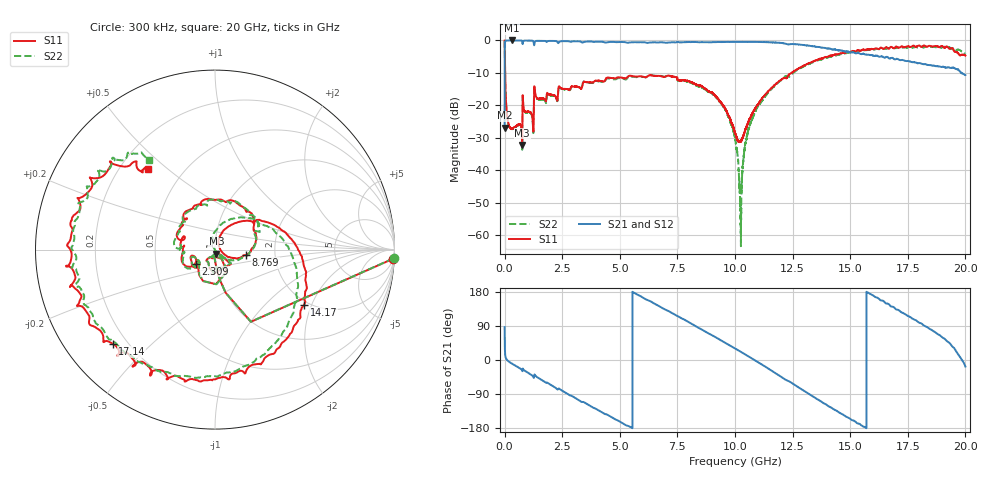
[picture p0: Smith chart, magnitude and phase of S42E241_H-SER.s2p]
! Created Wed Nov 25 22:07:44 2020
# khz S ma R 50
! 2 Port Network Data from SP1.SP block
! freq  magS11  angS11  magS21  angS21  magS12  angS12  magS22  angS22
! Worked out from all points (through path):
!   20001 points, 300 kHz to 20 GHz, reference 50 ohm
!   highest |S21| = -0.02 dB at 315.3 MHz (marker M1); lowest = -26.9 dB at 300 kHz (marker M2)
!   group delay of S21, straight-line fit = 97.6 ps
!   lowest |S11| = -32.2 dB at 763.3 MHz (marker M3), VSWR 1.05, Z = 50.8 - j2.36 ohm
!   |S11| at or under -10 dB: 20.12 MHz to 12.46 GHz (12.44 GHz wide, 199 % of centre)
!   |S22| runs from -63.4 to 0.0 dB; largest |S21 - S12| = 0.013
!   S11 on the Smith chart (normalised r, x): 300 kHz: 6, -38; 2.309 GHz: 0.80, -0.13; 8.769 GHz: 1.41, -0.09; 14.17 GHz: 1.90, -1.76; 17.14 GHz: 0.15, -0.38; 20 GHz: 0.32, +0.43
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300  0.9924 -3.0  0.04493 86.6  0.04459 86.7  0.9959 -2.8
103300  0.07189 -88.1  0.9948 0.2  0.9951 0.2  0.07176 -88.2
315300  0.04367 -96.5  0.9973 -9.4  0.9962 -9.5  0.04313 -96.8
763300  0.02454 -71.0  0.9798 -27.8  0.9799 -27.8  0.0206 -72.9
1370300  0.1345 -133.6  0.981 -43.4  0.9811 -43.4  0.1329 -131.8
2309300  0.1336 -144.3  0.9204 -77.8  0.9211 -77.8  0.1328 -140.0
3334300  0.1801 160.5  0.9443 -110.5  0.9444 -110.5  0.1818 175.0
5098300  0.266 109.1  0.946 -166.0  0.9459 -166.0  0.2586 103.0
6667300  0.2839 57.0  0.93 143.4  0.9295 143.4  0.2859 53.4
8769300  0.1744 -10.0  0.9425 72.9  0.9404 73.0  0.1684 -13.1
1.00003e7  0.03803 -17.7  0.9478 30.5  0.9476 30.6  0.03137 -55.8
1.02523e7  0.02776 31.7  0.9481 21.6  0.9468 21.6  0.00134 -154.0
1.05043e7  0.0471 65.4  0.9478 12.5  0.9488 12.5  0.03059 112.4
1.09863e7  0.102 67.4  0.946 -5.4  0.945 -5.3  0.09486 91.9
1.21103e7  0.2604 36.3  0.9018 -48.8  0.9016 -48.7  0.2641 41.3
1.33343e7  0.4625 -0.1  0.8155 -94.6  0.815 -94.6  0.4519 -10.2
1.41663e7  0.5834 -31.7  0.7371 -125.3  0.7321 -125.5  0.5631 -40.4
1.55413e7  0.7241 -83.4  0.6239 -174.6  0.6217 -174.2  0.6961 -86.4
1.66673e7  0.7459 -120.8  0.5355 147.5  0.5354 146.5  0.7577 -124.8
1.71353e7  0.7756 -137.4  0.4993 130.2  0.5002 129.2  0.7721 -141.3
1.84803e7  0.8205 177.7  0.4145 81.1  0.415 81.7  0.7914 173.1
2e7  0.5837 129.8  0.2906 -17.2  0.2906 -16.9  0.6269 126.4
